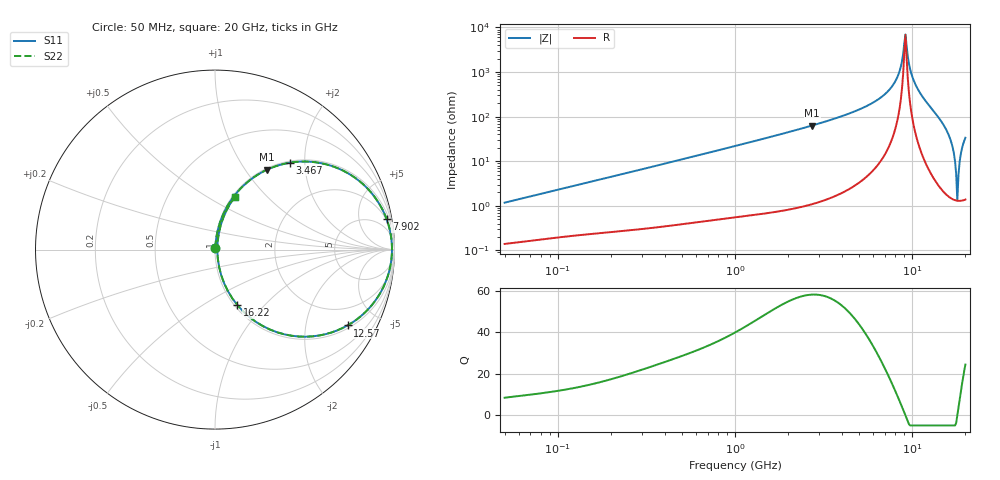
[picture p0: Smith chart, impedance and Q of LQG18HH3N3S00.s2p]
!Murata Part Number: LQG18HH3N3S00
!These Parameters are Measured in Series Mode Connection
!  o--[Z]--o
!Port1  Port2
!  o-------o
!Freq. Start=50[MHz] Stop=20[GHz], 401[Steps]
# Hz S RI R 50
!Freq.(Hz) S11(Real) S11(Imag) S21(Real) S21(Imag) S12(Real) S12(Imag) S22(Real) S22(Imag)
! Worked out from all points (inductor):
!   401 points, 50 MHz to 20 GHz, reference 50 ohm
!   read as one part in series: L = 3.69 nH near 51.52 MHz
!   highest Q = 58 at 2.728 GHz (marker M1), where L = 3.69 nH
!   self-resonance near 9.042 GHz
!   S11 on the Smith chart (normalised r, x): 50 MHz: 1.00, +0.02; 3.467 GHz: 1.03, +1.69; 7.902 GHz: 2, +11; 12.57 GHz: 1.12, -3.43; 16.22 GHz: 1.03, -0.72; 20 GHz: 1.03, +0.67
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5e7  0.00153 0.0117  0.9985 -0.0117  0.9985 -0.0117  0.00153 0.0117
1.364002e8  0.00316 0.0306  0.9968 -0.0306  0.9968 -0.0306  0.00316 0.0306
3.721004e8  0.00993 0.0809  0.9901 -0.0809  0.9901 -0.0809  0.00993 0.0809
1e9  0.0505 0.2068  0.9495 -0.2068  0.9495 -0.2068  0.0505 0.2068
2.728004e9  0.2892 0.4449  0.7108 -0.4449  0.7108 -0.4449  0.2892 0.4449
3.466789e9  0.4178 0.4844  0.5822 -0.4844  0.5822 -0.4844  0.4178 0.4844
5.598765e9  0.7516 0.419  0.2484 -0.419  0.2484 -0.419  0.7516 0.419
7.442007e9  0.9304 0.2281  0.0696 -0.2281  0.0696 -0.2281  0.9304 0.2281
7.901521e9  0.9561 0.1701  0.0439 -0.1701  0.0439 -0.1701  0.9561 0.1701
8.389408e9  0.9749 0.1057  0.0251 -0.1057  0.0251 -0.1057  0.9749 0.1057
8.907419e9  0.9849 0.0351  0.0151 -0.0351  0.0151 -0.0351  0.9849 0.0351
9.178299e9  0.986 -0.00233  0.014 0.00233  0.014 0.00233  0.986 -0.00233
1.034674e10  0.9569 -0.1642  0.0431 0.1642  0.0431 0.1642  0.9569 -0.1642
1.257102e10  0.7388 -0.4223  0.2612 0.4223  0.2612 0.4223  0.7388 -0.4223
1.438523e10  0.4266 -0.4799  0.5734 0.4799  0.5734 0.4799  0.4266 -0.4799
1.621653e10  0.1253 -0.31  0.8747 0.31  0.8747 0.31  0.1253 -0.31
1.696185e10  0.0511 -0.188  0.9489 0.188  0.9489 0.188  0.0511 -0.188
1.747767e10  0.0227 -0.0962  0.9773 0.0962  0.9773 0.0962  0.0227 -0.0962
1.800918e10  0.0128 -0.00105  0.9872 0.00105  0.9872 0.00105  0.0128 -0.00105
1.855685e10  0.0215 0.0926  0.9785 -0.0926  0.9785 -0.0926  0.0215 0.0926
1.912117e10  0.0471 0.1806  0.9529 -0.1806  0.9529 -0.1806  0.0471 0.1806
2e10  0.1114 0.2947  0.8886 -0.2947  0.8886 -0.2947  0.1114 0.2947
